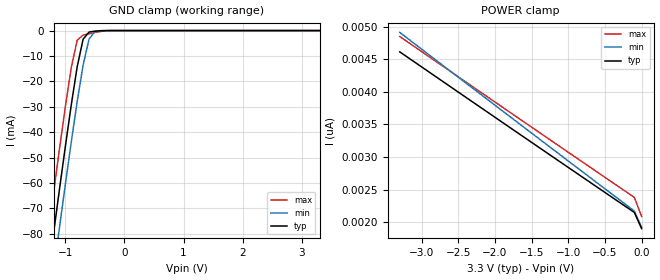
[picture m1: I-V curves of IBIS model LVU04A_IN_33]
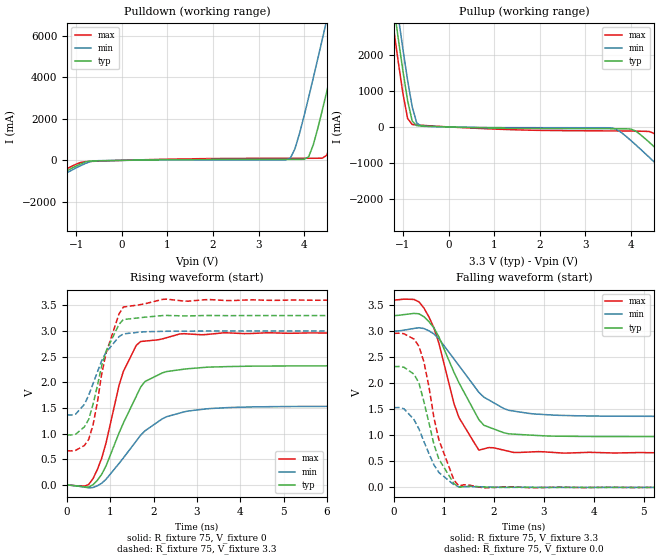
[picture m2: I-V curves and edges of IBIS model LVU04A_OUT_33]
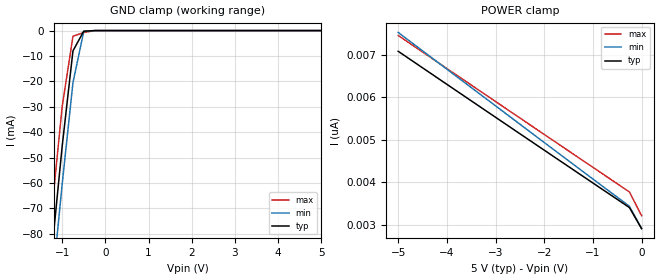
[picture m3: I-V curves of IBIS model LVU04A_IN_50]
| TEXAS INSTRUMENTS INCORPORATED
| Standard Linear and Logic Group
| IBIS Model of SN74LVU04A
| UNBUFFERED HEX INVERTER
| SOIC 14-pin (D), SOP 14-pin (NS), SSOP 14-pin (DB), TSSOP 14-pin (PW)
| and TVSOP 14-pin (DGV) Package
[IBIS Ver]   3.2
[Comment Char]  |_char
[File Name]   lvu04a.ibs
[File Rev]   2.0 H_die
[Date]   June 01, 2001
[Source]   Data created from HSPICE simulations at TI-SLL.
[Notes]   The following is an IBIS list for the LVU04A.
|   Please contact sllibis@ti.com with questions and
|   comments concerning SLL IBIS models.
[Disclaimer] Property of Texas Instruments Incorporated.  Unauthorized
   reproduction and/or distribution is strictly prohibited.
   This product is protected under copyright law.
   Created 2001, (C) Copyright 2001, Texas Instruments Inc.,
   All Rights Reserved.
   UNLESS THERE IS A SIGNED, WRITTEN AGREEMENT TO THE
   CONTRARY, TEXAS INSTRUMENTS ("TI") IS PROVIDING THE IBIS
   MODELS "AS IS" AND WITHOUT ANY WARRANTY, EXPRESSED OR
   IMPLIED.  TI assumes no liability for:
   1) the accuracy of the IBIS models provided to your
   company;
   2) the proper functioning of these IBIS Models in your
   design or for any resulting applications; or
   3) infringement of patents, copyrights or intellectual
   property rights resulting from your use of these IBIS
   models.
   TI provides IBIS Models as a service to our customers.
   You and your company shall not distribute, sell or give
   these models to anyone else without prior written
   permission from TI.
   TI reserves the right to make changes to our products or
   to discontinue any semiconductor product or service
   without notice, and advises our customers to obtain the
   latest version of relevant information to verify, before
   placing orders, that the information being relied on is
   current.
   Please be aware that your receipt and use of the IBIS
   information provided shall serve as acceptance of these
   terms and conditions.  If you do not accept these terms,
   you should return or destroy the IBIS models and any
   other accompanying information immediately.
|   Component LVU04A_D
[Component]   LVU04A_D
[Manufacturer]  Texas Instruments, Inc.
[Package]
|   typ   min   max
R_pkg   0.031   0.028   0.034
L_pkg   3.109nH   2.462nH   3.889nH
C_pkg   0.473pF   0.363pF   0.628pF
[Pin]   signal_name   model_name   R_pin   L_pin   C_pin
1   1A   LVU04A_IN   0.033   3.854nH   0.622pF
2   1Y   LVU04A_OUT   0.032   3.188nH   0.473pF
3   2A   LVU04A_IN   0.028   2.462nH   0.377pF
4   2Y   LVU04A_OUT   0.031   2.596nH   0.363pF
5   3A   LVU04A_IN   0.028   2.521nH   0.372pF
6   3Y   LVU04A_OUT   0.034   3.250nH   0.476pF
7   GND   GND   0.034   3.889nH   0.628pF
8   4Y   LVU04A_OUT   0.034   3.889nH   0.628pF
9   4A   LVU04A_IN   0.034   3.250nH   0.476pF
10   5Y   LVU04A_OUT   0.028   2.521nH   0.372pF
11   5A   LVU04A_IN   0.031   2.596nH   0.364pF
12   6Y   LVU04A_OUT   0.028   2.462nH   0.377pF
13   6A   LVU04A_IN   0.032   3.188nH   0.473pF
14   VCC   POWER   0.033   3.854nH   0.622pF
|   Component LVU04A_NS
[Component]   LVU04A_NS
[Manufacturer]  Texas Instruments, Inc
[Package]
|   typ   min   max
R_pkg   0.045   0.039   0.054
L_pkg   3.796nH   2.561nH   4.952nH
C_pkg   0.528pF   0.288pF   0.710pF
[Pin]   signal_name   model_name   R_pin   L_pin   C_pin
1   1A   LVU04A_IN   0.047   4.867nH   0.706pF
2   1Y   LVU04A_OUT   0.051   4.083nH   0.592pF
3   2A   LVU04A_IN   0.041   2.915nH   0.376pF
4   2Y   LVU04A_OUT   0.039   2.561nH   0.288pF
5   3A   LVU04A_IN   0.041   3.101nH   0.430pF
6   3Y   LVU04A_OUT   0.047   4.047nH   0.589pF
7   GND   GND   0.051   4.909nH   0.700pF
8   4Y   LVU04A_OUT   0.045   4.784nH   0.694pF
9   4A   LVU04A_IN   0.054   4.176nH   0.597pF
10   5Y   LVU04A_OUT   0.039   3.287nH   0.449pF
11   5A   LVU04A_IN   0.039   2.586nH   0.294pF
12   6Y   LVU04A_OUT   0.040   2.802nH   0.371pF
13   6A   LVU04A_IN   0.049   4.080nH   0.593pF
14   VCC   POWER   0.052   4.952nH   0.710pF
|   Component LVU04A_DB
[Component]   LVU04A_DB
[Manufacturer]  Texas Instruments, Inc.
[Package]
|   typ   min   max
R_pkg   0.044   0.041   0.046
L_pkg   3.551nH   3.258nH   3.927nH
C_pkg   0.402pF   0.360pF   0.421pF
[Pin]   signal_name   model_name   R_pin   L_pin   C_pin
1   1A   LVU04A_IN   0.046   3.927nH   0.408pF
2   1Y   LVU04A_OUT   0.044   3.587nH   0.421pF
3   2A   LVU04A_IN   0.041   3.289nH   0.398pF
4   2Y   LVU04A_OUT   0.042   3.258nH   0.360pF
5   3A   LVU04A_IN   0.041   3.286nH   0.403pF
6   3Y   LVU04A_OUT   0.044   3.586nH   0.421pF
7   GND   GND   0.046   3.927nH   0.408pF
8   4Y   LVU04A_OUT   0.046   3.927nH   0.408pF
9   4A   LVU04A_IN   0.044   3.586nH   0.421pF
10   5Y   LVU04A_OUT   0.041   3.286nH   0.403pF
11   5A   LVU04A_IN   0.043   3.258nH   0.360pF
12   6Y   LVU04A_OUT   0.041   3.289nH   0.398pF
13   6A   LVU04A_IN   0.044   3.587nH   0.421pF
14   VCC   POWER   0.046   3.927nH   0.408pF
|   Component LVU04A_PW
[Component]   LVU04A_PW
[Manufacturer]  Texas Instruments, Inc.
[Package]
|   typ   min   max
R_pkg   0.032   0.029   0.035
L_pkg   2.378nH   2.170nH   2.680nH
C_pkg   0.314pF   0.270pF   0.335pF
[Pin]   signal_name   model_name   R_pin   L_pin   C_pin
1   1A   LVU04A_IN   0.033   2.618nH   0.330pF
2   1Y   LVU04A_OUT   0.031   2.313nH   0.317pF
3   2A   LVU04A_IN   0.030   2.310nH   0.314pF
4   2Y   LVU04A_OUT   0.031   2.173nH   0.272pF
5   3A   LVU04A_IN   0.030   2.204nH   0.309pF
6   3Y   LVU04A_OUT   0.032   2.315nH   0.317pF
7   GND   GND   0.035   2.680nH   0.335pF
8   4Y   LVU04A_OUT   0.033   2.640nH   0.333pF
9   4A   LVU04A_IN   0.034   2.347nH   0.319pF
10   5Y   LVU04A_OUT   0.029   2.277nH   0.313pF
11   5A   LVU04A_IN   0.031   2.170nH   0.270pF
12   6Y   LVU04A_OUT   0.031   2.244nH   0.311pF
13   6A   LVU04A_IN   0.033   2.343nH   0.321pF
14   VCC   POWER   0.035   2.657nH   0.332pF
|   Component LVU04A_DGV
[Component]   LVU04A_DGV
[Manufacturer]  Texas Instruments, Inc.
[Package]
|   typ   min   max
R_pkg   0.035   0.020   0.045
L_pkg   2.499nH   2.077nH   2.966nH
C_pkg   0.361pF   0.305pF   0.416pF
[Pin]   signal_name   model_name   R_pin   L_pin   C_pin
1   1A   LVU04A_IN   0.027   2.717nH   0.373pF
2   1Y   LVU04A_OUT   0.037   2.434nH   0.398pF
3   2A   LVU04A_IN   0.034   2.200nH   0.316pF
4   2Y   LVU04A_OUT   0.020   2.077nH   0.309pF
5   3A   LVU04A_IN   0.030   2.147nH   0.305pF
6   3Y   LVU04A_OUT   0.042   2.580nH   0.408pF
7   GND   GND   0.039   2.921nH   0.385pF
8   4Y   LVU04A_OUT   0.033   2.841nH   0.380pF
9   4A   LVU04A_IN   0.042   2.611nH   0.410pF
10   5Y   LVU04A_OUT   0.038   2.331nH   0.329pF
11   5A   LVU04A_IN   0.026   2.223nH   0.319pF
12   6Y   LVU04A_OUT   0.034   2.259nH   0.313pF
13   6A   LVU04A_IN   0.045   2.681nH   0.416pF
14   VCC   POWER   0.042   2.966nH   0.386pF
[Model Selector]   LVU04A_IN
LVU04A_IN_33   3.3-V Vcc Input Model
LVU04A_IN_50   5.0-V Vcc Input Model
[Model Selector]   LVU04A_OUT
LVU04A_OUT_33   3.3-V Vcc Output Model
LVU04A_OUT_50   5.0-V Vcc Output Model
| Models and submodels in the file (4): LVU04A_IN_33 (Input), LVU04A_OUT_33 (Output), LVU04A_IN_50 (Input), LVU04A_OUT_50 (Output)
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|   Model LVU04A_IN_33
[Model]   LVU04A_IN_33
Model_type  Input
Polarity   Non-Inverting
Vinl = 0.66
Vinh = 2.64
| variable   typ   min   max
C_comp   2.51pf   1.88pf   3.14pf
[Temperature Range]   25   85   -40
[Voltage Range]   3.3   3.0   3.6
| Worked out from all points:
|   GND clamp passes 1 mA (typ) near -0.61 V on its own axis
[GND Clamp]
|   Voltage   I(typ)   I(min)   I(max)
-3.3V     -460.4mA   -474.6mA   -445.4mA
-1.3V     -97.49mA   -112.5mA   -81.51mA
-1.2V     -79.93mA   -94.98mA   -63.94mA
-1.1V     -62.59mA   -77.62mA   -46.67mA
-1V       -45.6mA    -60.54mA   -29.97mA
-900mV    -29.25mA   -43.87mA   -14.58mA
-800mV    -14.28mA   -27.95mA   -3.811mA
-700mV    -3.418mA   -13.61mA   -1.784mA
-600mV    -581.1uA   -3.398mA   -1.247mA
-500mV    -232.6uA   -352.5uA   -758.6uA
-400mV    -58.12uA   -21.94uA   -324.1uA
3.3V      1.902nA    2.343nA    1.692nA
[POWER Clamp]
|   Voltage   I(typ)   I(min)   I(max)
-3.3V     4.612nA    4.91nA     4.847nA
-1.6V     3.301nA    3.451nA    3.534nA
-100mV    2.151nA    2.173nA    2.382nA
0V        1.902nA    1.921nA    2.089nA
|   Model LVU04A_OUT_33
[Model]   LVU04A_OUT_33
Model_type  Output
Polarity   Inverting
Vmeas = 1.65v
Cref = 15pf
| variable   typ   min   max
C_comp   6.50pf   4.88pf   8.13pf
[Temperature Range]   25   85   -40
[Voltage Range]   3.3   3.0   3.6
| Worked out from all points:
|   slope of the pulldown table from 0 to 0.495 V, typ, clamps not added: 27.3 ohm
|   slope of the pullup table from 0 to 0.495 V, typ, clamps not added: 28.4 ohm
|   rising waveform, R_fixture 75, V_fixture 0: 20-80 % time 728ps typ, 1ns min, 569ps max; typ from 0 V to 2.32 V
|   falling waveform, R_fixture 75, V_fixture 3.3: 20-80 % time 697ps typ, 835ps min, 540ps max; typ from 3.3 V to 0.976 V
|   rising waveform, R_fixture 75, V_fixture 3.3: 20-80 % time 476ps typ, 520ps min, 457ps max; typ from 0.976 V to 3.3 V
|   falling waveform, R_fixture 75, V_fixture 0.0: 20-80 % time 408ps typ, 443ps min, 416ps max; typ from 2.32 V to 0 V
[Pulldown]
|   Voltage   I(typ)   I(min)   I(max)
-3.3V     -3.044A    -3.131A    -2.953A
-800mV    -79.06mA   -150.8mA   -61.66mA
3.7V      47.05mA    113.5mA    99.69mA
3.8V      47.15mA    562mA      100.1mA
4.1V      172.6mA    3.031A     101.1mA
4.2V      734.8mA    3.949A     101.6mA
4.4V      2.417A     5.828A     105.3mA
4.5V      3.333A     6.781A     252.7mA
4.6V      4.268A     7.74A      912.6mA
4.8V      6.173A     9.671A     2.68A
5.2V      10.05A     13.57A     6.497A
6.6V      23.82A     27.35A     20.27A
[Pullup]
|   Voltage   I(typ)   I(min)   I(max)
-3.3V     23.82A     24.39A     23.24A
-1.2V     3.332A     3.949A     2.678A
-1.1V     2.416A     3.031A     1.765A
-900mV    732.4mA    1.296A     235.4mA
-800mV    165.4mA    561.2mA    67.92mA
-700mV    36.78mA    110.7mA    56.21mA
-600mV    27.55mA    21.73mA    47.27mA
3.6V      -50.35mA   -30.84mA   -111.4mA
4.1V      -112.8mA   -493.8mA   -116.9mA
4.5V      -541.7mA   -963.7mA   -176.5mA
6V        -2.354A    -2.784A    -1.949A
6.6V      -3.09A     -3.519A    -2.685A
[Ramp]
| variable   typ   min   max
dV/dt_r  1.3925E+00/6.7179E-10  9.1965E-01/9.9075E-10  1.7765E+00/5.5832E-10
dV/dt_f  1.4199E+00/6.3609E-10  1.0213E+00/8.4332E-10  1.7743E+00/5.2859E-10
R_load = 75
[Rising Waveform]
R_fixture = 75
V_fixture = 0
|   Time   V(typ)   V(min)   V(max)
0s        0V         0V         0V
400ps     -36.3mV    -39.81mV   -21.25mV
600ps     6.683mV    -47.82mV   126.5mV
900ps     373.6mV    112.3mV    820.2mV
1.3ns     1.207V     527.5mV    2.212V
1.6ns     1.733V     860.2mV    2.723V
1.8ns     2.016V     1.056V     2.803V
2.6ns     2.244V     1.401V     2.941V
5.2ns     2.319V     1.529V     2.955V
25ns      2.321V     1.533V     2.96V
[Falling Waveform]
R_fixture = 75
V_fixture = 3.3
V_fixture_min = 3.0
V_fixture_max = 3.6
|   Time   V(typ)   V(min)   V(max)
0s        3.3V       3V         3.6V
400ps     3.343V     3.054V     3.612V
600ps     3.28V      3.052V     3.447V
900ps     2.891V     2.854V     2.769V
1.2ns     2.214V     2.47V      1.616V
1.3ns     2.013V     2.342V     1.344V
1.7ns     1.301V     1.826V     715.9mV
2.3ns     1.029V     1.481V     693.4mV
3.7ns     980.2mV    1.376V     667.3mV
25ns      976mV      1.365V     666mV
[Rising Waveform]
R_fixture = 75
V_fixture = 3.3
V_fixture_min = 3.0
V_fixture_max = 3.6
|   Time   V(typ)   V(min)   V(max)
0s        976mV      1.365V     666mV
200ps     990.2mV    1.382V     676.6mV
500ps     1.279V     1.75V      890.8mV
600ps     1.573V     1.974V     1.172V
800ps     2.324V     2.422V     2.163V
900ps     2.607V     2.584V     2.566V
1.2ns     3.131V     2.889V     3.332V
1.3ns     3.223V     2.944V     3.466V
2.2ns     3.299V     2.993V     3.614V
25ns      3.3V       3V         3.6V
[Falling Waveform]
R_fixture = 75
V_fixture = 0.0
|   Time   V(typ)   V(min)   V(max)
0s        2.321V     1.533V     2.96V
200ps     2.31V      1.512V     2.952V
400ps     2.176V     1.305V     2.85V
500ps     2.006V     1.123V     2.712V
600ps     1.646V     882.2mV    2.411V
800ps     827.5mV    433.9mV    1.34V
900ps     541.8mV    286.6mV    913.5mV
1.2ns     74.21mV    50.6mV     142.1mV
1.3ns     2.446mV    11.5mV     25.97mV
25ns      0V         0V         0V
|   Model LVU04A_IN_50
[Model]   LVU04A_IN_50
Model_type  Input
Polarity   Non-Inverting
Vinl = 1.0
Vinh = 4.0
| variable   typ   min   max
C_comp   2.51pf   1.88pf   3.14pf
[Temperature Range]   25   85   -40
[Voltage Range]   5.0   4.5   5.5
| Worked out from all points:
|   GND clamp passes 1 mA (typ) near -0.52 V on its own axis
[GND Clamp]
|   Voltage   I(typ)   I(min)   I(max)
-5V       -772.7mA   -786.5mA   -758.1mA
-1.5V     -133mA     -148mA     -117.2mA
-1.25V    -88.68mA   -103.7mA   -72.7mA
-1V       -45.6mA    -60.54mA   -29.97mA
-750mV    -7.993mA   -20.49mA   -2.232mA
-500mV    -232.6uA   -352.5uA   -758.6uA
-250mV    -2.633nA   -182.1nA   -26.9uA
5V        2.904nA    3.644nA    2.541nA
[POWER Clamp]
|   Voltage   I(typ)   I(min)   I(max)
-5V       7.079nA    7.524nA    7.451nA
-2.5V     5.139nA    5.363nA    5.509nA
-250mV    3.401nA    3.43nA     3.769nA
0V        2.904nA    2.91nA     3.209nA
